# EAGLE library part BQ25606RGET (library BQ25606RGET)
Stand Alone Single Cell 3-A Fast Charger with High Input Voltage and Power Path Source: Datasheet
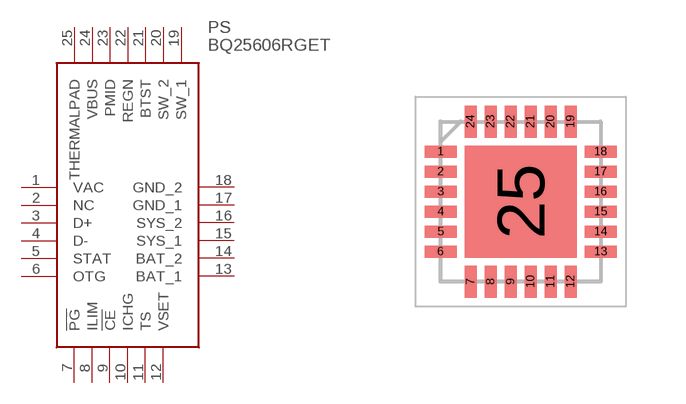
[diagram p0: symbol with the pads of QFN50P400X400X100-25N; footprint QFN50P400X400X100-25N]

Designator prefix PS

## BQ25606RGET (Description: Stand Alone Single Cell 3-A Fast Charger with High Input Voltage and Power Path; Height: 1mm; Manufacturer_Name: Texas Instruments; Manufacturer_Part_Number: BQ25606RGET; Mouser2_Part_Number: 595-BQ25606RGET; Mouser2_Price-Stock: https://www.mouser.com/Search/Refine.aspx?Keyword=595-BQ25606RGET)  [QFN50P400X400X100-25N]
1  VAC  in
2  NC  nc
3  D+
4  D-
5  STAT  out
6  OTG  in
7  !PG  out
8  ILIM  in
9  !CE  in
10  ICHG  in
11  TS  in
12  VSET  in
13  BAT_1  pwr
14  BAT_2  pwr
15  SYS_1  pwr
16  SYS_2  pwr
17  GND_1  pwr
18  GND_2  pwr
19  SW_1  pwr
20  SW_2  pwr
21  BTST  pwr
22  REGN  pwr
23  PMID  pwr
24  VBUS  pwr
25  THERMALPAD  pwr

## Footprint QFN50P400X400X100-25N (pad centres in mm)
VQFN-24
smd 0.8 x 0.3: 1 -2,1.25; 2 -2,0.75; 3 -2,0.25; 4 -2,-0.25; 5 -2,-0.75; 6 -2,-1.25; 13 2,-1.25; 14 2,-0.75; 15 2,-0.25; 16 2,0.25; 17 2,0.75; 18 2,1.25
smd 0.3 x 0.8: 7 -1.25,-2; 8 -0.75,-2; 9 -0.25,-2; 10 0.25,-2; 11 0.75,-2; 12 1.25,-2; 19 1.25,2; 20 0.75,2; 21 0.25,2; 22 -0.25,2; 23 -0.75,2; 24 -1.25,2
smd 2.8 x 2.8: 25 0,0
